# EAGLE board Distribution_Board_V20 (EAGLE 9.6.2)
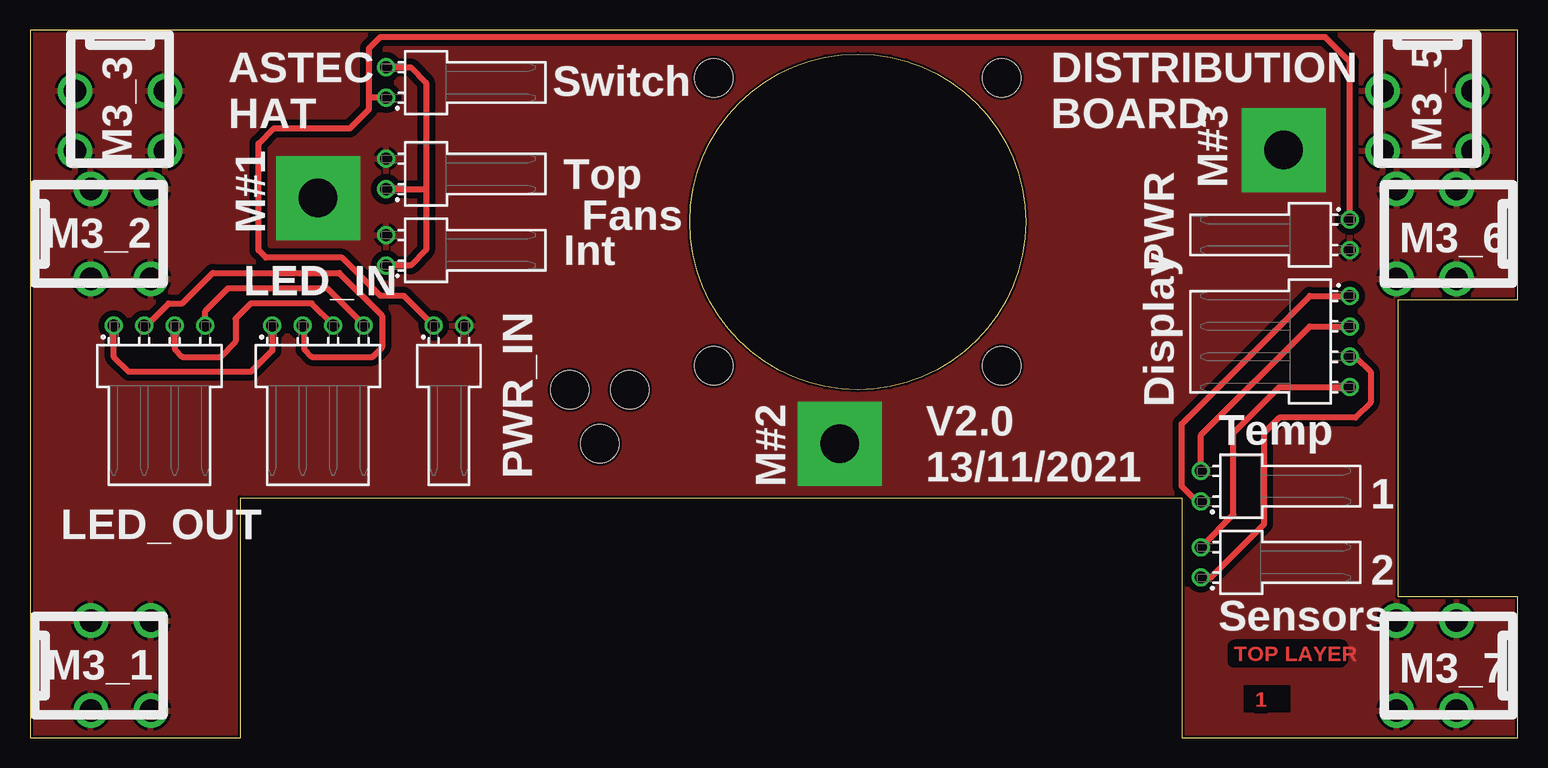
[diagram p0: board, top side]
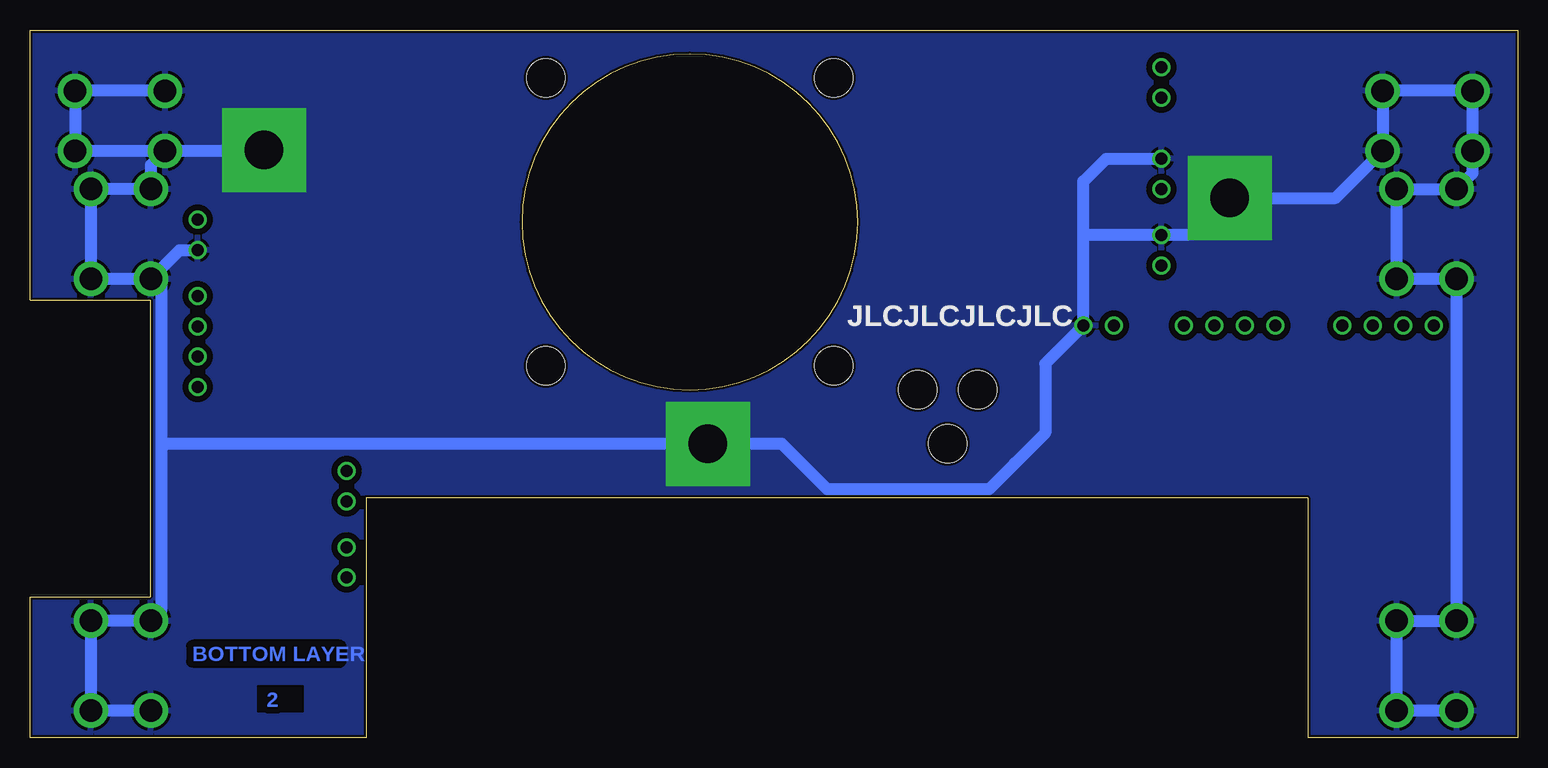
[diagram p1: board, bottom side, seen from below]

Size 124 x 59 mm. Coordinates in mm from the lower left corner, seen from the top.
Outline: 0,0 17.5,0 17.5,20 96,20 96,0 124,0 124,11.75 114,11.75 114,36.5 124,36.5 124,59 0,59 0,0
Outline: 55,43 arc-180 83,43 arc-180 55,43
Copper layers (1*16): Top 0.035mm / dielectric 1.5mm / Bottom 0.035mm
Design rules "JLCPCB_2alyer": minimum track width 5mil, minimum drill 0.2mm, track to track 5mil, track to pad 0.2mm, pad to pad 0.2mm, via to via 0.2mm, smd to smd 5mil, copper to edge 0.2mm, drill to drill 0.5mm, minimum pad ring 0.13mm, minimum via ring 0.13mm, stop-mask expansion 0.05mm, vias tented up to drill 0mil, thermal gap 10mil
Net classes: 1 Versorgung: width 1 mm, drill 0.6 mm, clearance 0.5 mm
Holes 3.2 mm at 57,55 57,31 81,55 81,31 47.5,24.5 45,29 50,29
tRestrict: 12 lines
bRestrict: 12 lines
Milling: 2 lines

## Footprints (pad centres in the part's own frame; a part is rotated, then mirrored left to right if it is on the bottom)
61900411021 = drill 1: 1 -3.81,3.35; 2 -1.27,3.35; 3 1.27,3.35; 4 3.81,3.35
61900211021 = drill 1: 1 -1.27,3.35; 2 1.27,3.35
KEYSTONE_7761_PCB_SCREW_M3 = drill 1.9: P$1 5.08,-3.75; P$2 5.08,3.75; P$3 10.08,3.75; P$4 10.08,-3.75
M-PAD_M3(POLYGON) = drill 3.2 pad 7 square: P$1 0,0

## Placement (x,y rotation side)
J1  61900411021  [61900411021]  10.79,31 0 top
J2  61900411021  [61900411021]  24,31 0 top
J3  61900211021  [61900211021]  106.68,41.91 270 top
J4  61900411021  [61900411021]  106.68,33.02 270 top
J5  61900211021  [61900211021]  100.97,14.61 90 top
J6  61900211021  [61900211021]  100.97,20.95 90 top
J7  61900211021  [61900211021]  34.92,31 0 top
J8  61900211021  [61900211021]  33.02,46.99 90 top
J9  61900211021  [61900211021]  33.02,54.61 90 top
J10  61900211021  [61900211021]  33.02,40.64 90 top
M3_1  KEYSTONE_7761_PCB_SCREW_M3  [KEYSTONE_7761_PCB_SCREW_M3]  0,6 0 top
M3_2  KEYSTONE_7761_PCB_SCREW_M3  [KEYSTONE_7761_PCB_SCREW_M3]  0,42 0 top
M3_3  KEYSTONE_7761_PCB_SCREW_M3  [KEYSTONE_7761_PCB_SCREW_M3]  7.5,59 270 top
M3_5  KEYSTONE_7761_PCB_SCREW_M3  [KEYSTONE_7761_PCB_SCREW_M3]  116.5,59 270 top
M3_6  KEYSTONE_7761_PCB_SCREW_M3  [KEYSTONE_7761_PCB_SCREW_M3]  124,42 180 top
M3_7  KEYSTONE_7761_PCB_SCREW_M3  [KEYSTONE_7761_PCB_SCREW_M3]  124,6 180 top
M#1  M-PAD_M3(POLYGON)  [M-PAD_M3(POLYGON)]  24,45 0 top
M#2  M-PAD_M3(POLYGON)  [M-PAD_M3(POLYGON)]  67.5,24.5 0 top
M#3  M-PAD_M3(POLYGON)  [M-PAD_M3(POLYGON)]  104.5,49 0 top

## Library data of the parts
J1 J2 J4 = Eagle_WR-WTB (rev20a); CONTACT-RESISTANCE: 20mOhm; DATASHEET-URL: https://www.we-online.com/catalog/datasheet/61900411021.pdf; GENDER: Male; L: 10.16mm; MOUNT: THT; PACKAGING: Bag; PART-NUMBER: 61900411021; PCB-CABLE-PANEL: PCB; PINS: 4; PITCH: 2.54mm; TOL-R: max.; TYPE: Right Angled Bottom Locking; USE-WITH: WR-WTB 2.54 mm Female Terminal Housing; WORKING-VOLTAGE: 250V(AC)
J3 J5-J10 = Eagle_WR-WTB (rev20a); CONTACT-RESISTANCE: 20mOhm; DATASHEET-URL: https://www.we-online.com/catalog/datasheet/61900211021.pdf; GENDER: Male; L: 5.08mm; MOUNT: THT; PACKAGING: Bag; PART-NUMBER: 61900211021; PCB-CABLE-PANEL: PCB; PINS: 2; PITCH: 2.54mm; TOL-R: max.; TYPE: Right Angled Bottom Locking; USE-WITH: WR-WTB 2.54 mm Female Terminal Housing; WORKING-VOLTAGE: 250V(AC)
M3_1-M3_3 M3_5-M3_7 M#1-M#3 = Antec-Hood

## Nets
GND [Versorgung]: J3.2 J7.2 J8.2 J10.2 M3_1.P$1 M3_1.P$2 M3_1.P$3 M3_1.P$4 M3_2.P$1 M3_2.P$2 M3_2.P$3 M3_2.P$4 M3_3.P$1 M3_3.P$2 M3_3.P$3 M3_3.P$4 M3_5.P$1 M3_5.P$2 M3_5.P$3 M3_5.P$4 M3_6.P$1 M3_6.P$2 M3_6.P$3 M3_6.P$4 M3_7.P$1 M3_7.P$2 M3_7.P$3 M3_7.P$4 M#1.P$1 M#2.P$1 M#3.P$1
N$1: J1.1 J2.1
N$2: J1.2 J2.2
N$3: J4.2 J6.2
N$4: J4.3 J5.1
N$5: J4.4 J5.2
N$6: J4.1 J6.1
N$7: J8.1 J9.2 J10.1
N$11: J3.1 J7.1 J9.1
N$12: J1.3 J2.3
N$14: J1.4 J2.4

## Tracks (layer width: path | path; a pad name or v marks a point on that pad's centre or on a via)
GND
  Bottom 1: M3_1.P$1 M3_1.P$4 M3_1.P$3 M3_1.P$2 M3_2.P$1 M3_2.P$4 M3_2.P$3 M3_2.P$2 3.75,47.08 M3_3.P$4 M3_3.P$1 M3_3.P$2 M3_3.P$3 | M3_5.P$1 M3_5.P$2 M3_5.P$3 M3_5.P$4 113.92,47.75 M3_6.P$4 M3_6.P$1 M3_6.P$2 | M3_7.P$3 M3_7.P$2 M3_7.P$1 M3_7.P$4 | 41.91,22.86 44.07,20.7 57.53,20.7 61.33,24.5 M#2.P$1 112.66,24.5 113.03,24.13 | M3_6.P$3 111.53,40.64 J3.2 | M#1.P$1 27.09,41.91 J10.2
  Bottom 1.016: M3_5.P$4 104.58,48.92 M#3.P$1 | M#1.P$1 15.17,45 M3_3.P$3 | M3_7.P$4 113.03,10.64 113.03,24.13 113.03,38.1 113.18,38.25 M3_6.P$3 M3_6.P$2 | 36.2,41.91 J7.2 39.37,31.18 39.37,25.4 41.91,22.86 | 36.2,41.91 36.2,46.35 34.29,48.26 J8.2 | J10.2 36.2,41.91
  pour Bottom: -3.81,62.23 -3.81,-5.08 129.54,-5.08 130.81,-3.81 130.81,63.5 -2.54,63.5
  pour Top: -5.08,62.23 -5.08,-2.54 -2.54,-5.08 129.54,-5.08 129.54,62.23 125.73,66.04 -1.27,66.04
N$1
  Top 0.508: J1.1 6.99,31.75 8.26,30.48 18.41,30.48 20.19,32.26 J2.1
N$2
  Top 0.508: J1.2 9.71,34.35 11.56,36.2 12.7,36.2 15.24,38.73 25.78,38.73 29.34,35.18 29.34,32.51 28.57,31.75 23.5,31.75 22.86,32.38 22.86,34.22 J2.2
N$3
  Top 0.508: J6.2 97.61,25.23 106.68,34.29 J4.2
N$4
  Top 0.508: J4.3 110.49,31.75 111.76,30.48 111.76,27.94 110.49,26.67 104.14,26.67 102.87,25.4 102.87,17.78 98.42,13.34 J5.1
N$5
  Top 0.508: J5.2 100.33,18.59 100.33,25.4 104.14,29.21 J4.4
N$6
  Top 0.508: J6.1 97.28,19.68 96.01,20.95 96.01,26.16 106.68,36.83 J4.1
N$7
  Top 0.508: J9.2 31.75,55.88 33.02,54.61 33.02,45.72 | J10.1 31.75,39.37 33.02,40.64 33.02,45.72 | J8.1 33.02,45.72
N$11
  Top 0.508: J7.1 31.18,36.83 29.21,36.83 26.04,40.01 19.68,40.01 19.05,40.64 19.05,49.53 20.32,50.8 26.67,50.8 28.25,52.38 28.25,53.34 | 28.25,53.34 28.25,57.46 29.21,58.42 107.95,58.42 110.03,56.34 J3.1 | J9.1 28.25,53.34
N$12
  Top 0.508: J2.3 25.27,34.42 23.5,36.2 18.41,36.2 17.14,34.92 17.14,33.02 15.88,31.75 12.7,31.75 12.06,32.38 J1.3
N$14
  Top 0.508: J1.4 14.61,35.56 16.51,37.47 24.77,37.47 27.81,34.42 J2.4

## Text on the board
Top: TOP LAYER | 1
Bottom: BOTTOM LAYER | 2
tPlace: Switch | ASTEC / HAT | DISTRIBUTION / BOARD | Top | Fans | Int | PWR | LED_IN | Display | Temp | PWR_IN | V2.0 / 13/11/2021 | 1 | LED_OUT | 2 | Sensors
bPlace: JLCJLCJLCJLC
